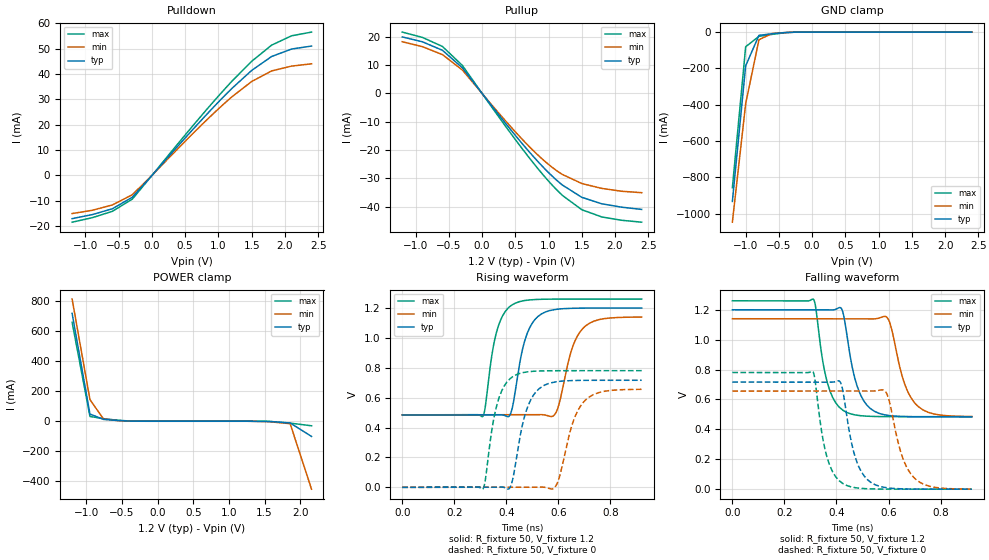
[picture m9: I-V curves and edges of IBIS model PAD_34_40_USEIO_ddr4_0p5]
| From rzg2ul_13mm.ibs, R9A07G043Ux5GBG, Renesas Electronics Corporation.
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[Model] PAD_34_40_USEIO_ddr4_0p5
Model_type I/O
Polarity   Non-Inverting
Vinl = 0.5070
Vinh = 0.6930
Vmeas= 0.600
| Capacitance   typ   min   max
C_comp   2.102e-12   2.013e-12   2.214e-12
[Model Spec]
| Subparameter   typ   min   max
Vmeas   0.600   0.570   0.630
Vinh   0.6930   0.6630   0.7230
Vinl   0.5070   0.4770   0.5370
| Variables   typ   min   max
[GND Clamp Reference]   0   0   0
[POWER Clamp Reference]   1.2   1.14   1.26
[Pulldown Reference]   0   0   0
[Pullup Reference]   1.2   1.14   1.26
[Temperature Range]   25   125   -40
[Voltage Range]   1.2   1.14   1.26
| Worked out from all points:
|   slope of the pulldown table from 0 to 0.18 V, typ, clamps not added: 33.6 ohm
|   slope of the pullup table from 0 to 0.18 V, typ, clamps not added: 33.2 ohm
|   GND clamp passes 1 mA (typ) near -0.30 V on its own axis
|   POWER clamp passes 1 mA (typ) near -0.38 V on its own axis
|   rising waveform, R_fixture 50, V_fixture 1.2: 20-80 % time 53.8ps typ, 61.1ps min, 48.1ps max; typ from 0.484 V to 1.2 V
|   rising waveform, R_fixture 50, V_fixture 0: 20-80 % time 56.3ps typ, 65.4ps min, 50ps max; typ from 0 V to 0.717 V
|   falling waveform, R_fixture 50, V_fixture 1.2: 20-80 % time 55.6ps typ, 64.6ps min, 50.6ps max; typ from 1.2 V to 0.484 V
|   falling waveform, R_fixture 50, V_fixture 0: 20-80 % time 55.2ps typ, 63.4ps min, 49.6ps max; typ from 0.716 V to 0 V
[GND Clamp]
| Voltage   I(typ)   I(min)   I(max)
-1.2V     -932.7mA   -1.047A    -857.4mA
-1V       -185.5mA   -394.3mA   -80.64mA
-800mV    -17.89mA   -41.9mA    -23.65mA
-600mV    -9.04mA    -7.411mA   -12.44mA
-400mV    -2.454mA   -2.378mA   -3.185mA
2.4V      0A         0A         0A
[POWER Clamp]
| Voltage   I(typ)   I(min)   I(max)
-1.2V     719.7mA    815.2mA    660.1mA
-950mV    48.1mA     144.6mA    32.07mA
-760mV    12.41mA    14.91mA    17.11mA
-360mV    527.4uA    791.2uA    575.5uA
1.26V     -115.5nA   -12.89uA   -796.6pA
1.56V     -1.53mA    -2.776mA   -549.4uA
1.86V     -11.39mA   -16.33mA   -12.44mA
2.16V     -101.5mA   -453.2mA   -30.39mA
[Pulldown]
| Voltage   I(typ)   I(min)   I(max)
-1.2V     -17mA      -15mA      -18.4mA
-895mV    -15.4mA    -13.7mA    -16.61mA
-595mV    -13.11mA   -11.61mA   -14.12mA
-295mV    -8.579mA   -7.589mA   -9.313mA
450mV     13.33mA    12.15mA    14.39mA
905mV     26.33mA    23.91mA    28.46mA
1.21V     34.48mA    31.15mA    37.34mA
1.5V      41.4mA     37.03mA    44.99mA
1.8V      46.89mA    41.2mA     51.36mA
2.1V      49.82mA    43.1mA     55.04mA
2.4V      51mA       44mA       56.5mA
[Pullup]
| Voltage   I(typ)   I(min)   I(max)
-1.2V     19.9mA     18.2mA     21.6mA
-895mV    18.16mA    16.46mA    19.71mA
-595mV    15.18mA    13.66mA    16.52mA
-295mV    8.993mA    8.219mA    9.816mA
300mV     -8.991mA   -8.272mA   -9.855mA
650mV     -18.99mA   -17.31mA   -20.9mA
955mV     -26.87mA   -24.16mA   -29.72mA
1.21V     -32.34mA   -28.6mA    -35.99mA
1.5V      -36.63mA   -31.77mA   -41mA
1.8V      -38.92mA   -33.49mA   -43.55mA
2.1V      -40.11mA   -34.5mA    -44.73mA
2.4V      -40.9mA    -35mA      -45.4mA
[Ramp]
dV/dt_r   0.4296/5.383e-11   0.3925/6.114e-11   0.4649/4.808e-11
dV/dt_f   0.4298/5.520e-11   0.3935/6.340e-11   0.4682/4.958e-11
R_load= 50
[Rising Waveform]
R_fixture = 50
V_fixture = 1.2
V_fixture_min = 1.14
V_fixture_max = 1.26
| Time   V(typ)   V(min)   V(max)
0s        484mV      485.3mV    485.2mV
310ps     484mV      485.3mV    475.3mV
356ps     484.2mV    485.3mV    993.5mV
409ps     473.4mV    485.3mV    1.203V
481ps     1.034V     485.3mV    1.253V
577ps     1.187V     475mV      1.26V
602ps     1.193V     553.1mV    1.26V
654ps     1.198V     936.4mV    1.26V
692ps     1.199V     1.06V      1.26V
920ps     1.2V       1.14V      1.26V
[Rising Waveform]
R_fixture = 50
V_fixture = 0
V_fixture_min = 0
V_fixture_max = 0
| Time   V(typ)   V(min)   V(max)
0s        88.32nV    3.707uV    12.95nV
310ps     -1.399uV   3.487uV    -10.64mV
358ps     303.7uV    3.223uV    511.8mV
410ps     -9.847mV   17.09uV    719.6mV
483ps     544.1mV    -82.17uV   773.4mV
579ps     702.1mV    -9.723mV   780.4mV
604ps     709.3mV    68.85mV    780.6mV
656ps     714.7mV    436mV      780.7mV
696ps     716mV      569.3mV    780.8mV
920ps     716.6mV    655.9mV    780.8mV
[Falling Waveform]
R_fixture = 50
V_fixture = 1.2
V_fixture_min = 1.14
V_fixture_max = 1.26
| Time   V(typ)   V(min)   V(max)
0s        1.2V       1.14V      1.26V
311ps     1.2V       1.14V      1.27V
365ps     1.199V     1.14V      711.5mV
417ps     1.212V     1.14V      539mV
464ps     788.6mV    1.14V      499.6mV
492ps     632.5mV    1.14V      491.5mV
590ps     495.8mV    1.154V     485.2mV
660ps     485.6mV    714.2mV    484.8mV
700ps     484.3mV    578.1mV    484.8mV
920ps     483.7mV    485.9mV    484.8mV
[Falling Waveform]
R_fixture = 50
V_fixture = 0
V_fixture_min = 0
V_fixture_max = 0
| Time   V(typ)   V(min)   V(max)
0s        716.3mV    656.3mV    780.4mV
309ps     716.3mV    656.3mV    786.5mV
358ps     716mV      656.3mV    251mV
411ps     722.8mV    656.2mV    55.78mV
484ps     157.3mV    656.1mV    6.923mV
580ps     13mV       663.2mV    405.7uV
602ps     7.334mV    595.6mV    215.6uV
652ps     2.069mV    222.3mV    57.66uV
694ps     642.2uV    84.23mV    12.64uV
920ps     1.101uV    452.2uV    28.75nV
[Add Submodel]
| Submodel Name Mode
PAD_34_40_0p5_T Non-Driving
